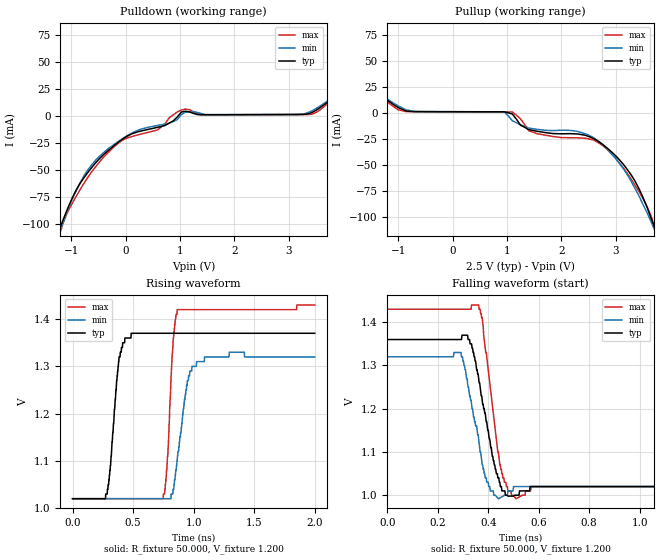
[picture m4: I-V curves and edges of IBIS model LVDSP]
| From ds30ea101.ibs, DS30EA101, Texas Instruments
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|   Model LVDSP
[Model]  LVDSP
Model_type Output
Polarity   Non-Inverting
Vmeas =  1.2V
Rref =   50.0000
Vref =   1.20V
C_comp   417fF   403fF   425fF
[Temperature Range]   25.0000   85.0000   -40.0000
[Voltage Range]   2.5000V   2.3750V   2.6250V
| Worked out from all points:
|   slope of the pulldown table from 0 to 0.375 V, typ, clamps not added: 55.7 ohm
|   slope of the pullup table from 0 to 0.375 V, typ, clamps not added: 8.04 kohm
|   rising waveform, R_fixture 50.000, V_fixture 1.200: 20-80 % time 66ps typ, 94ps min, 47.2ps max; typ from 1.02 V to 1.37 V
|   falling waveform, R_fixture 50.000, V_fixture 1.200: 20-80 % time 64.8ps typ, 56ps min, 51.2ps max; typ from 1.36 V to 1.02 V
[Pulldown]
|Voltage   I(typ)   I(min)   I(max)
-2.5V     -573mA     -566mA     -612mA
-1.225V   -106mA     -109mA     -111mA
-925mV    -69.8mA    -70.7mA    -75.7mA
-700mV    -52.5mA    -50mA      -57mA
-475mV    -39.1mA    -37mA      -42.1mA
-100mV    -22.9mA    -22.3mA    -23.7mA
575mV     -10.5mA    -8.8mA     -13mA
1.025V    3.82mA     1.52mA     5.6mA
3.2V      1.52mA     1.62mA     1.43mA
3.5V      5.37mA     7mA        3.26mA
4.025V    25.9mA     25.5mA     26.5mA
5V        72.8mA     66.5mA     81.9mA
[Pullup]
|Voltage   I(typ)   I(min)   I(max)
-2.5V     72.79mA    66.54mA    81.87mA
-1V       5.372mA    6.997mA    3.261mA
-700mV    1.519mA    1.612mA    1.433mA
950mV     1.29mA     1.332mA    1.182mA
1.1V      -808.5uA   -7.312mA   1.164mA
1.4V      -15.8mA    -14.32mA   -16.88mA
2.45V     -21.31mA   -19.9mA    -24.13mA
2.75V     -29.63mA   -29.55mA   -30.62mA
3.2V      -53.08mA   -57.94mA   -56.71mA
3.5V      -80.59mA   -87.38mA   -81.84mA
3.73V     -111.6mA   -113.6mA   -111.5mA
5V        -569.3mA   -565mA     -608.3mA
[Ramp]
| variable   typ   min   max
dV/dt_r   211.801m/65.502p   201.598m/87.621p   224.397m/48.781p
dV/dt_f   209.399m/58.418p   193.803m/65.933p   224.396m/46.560p
R_load = 50.00
[Rising Waveform]
R_fixture = 50.000
V_fixture = 1.200
V_fixture_min = 1.100
V_fixture_max = 1.300
|  time   V(typ)   V(min)   V(max)
0s        1.02V      1.02V      1.02V
286ps     1.03V      1.02V      1.02V
384ps     1.32V      1.02V      1.02V
484ps     1.37V      1.02V      1.02V
760ps     1.37V      1.02V      1.03V
832ps     1.37V      1.04V      1.36V
864ps     1.37V      1.1V       1.42V
948ps     1.37V      1.27V      1.42V
1.024ns   1.37V      1.31V      1.42V
2ns       1.37V      1.32V      1.43V
[Falling Waveform]
R_fixture = 50.000
V_fixture = 1.200
V_fixture_min = 1.100
V_fixture_max = 1.300
|  time   V(typ)   V(min)   V(max)
0s        1.36V      1.32V      1.43V
292ps     1.36V      1.33V      1.43V
334ps     1.35V      1.21V      1.44V
362ps     1.27V      1.13V      1.44V
376ps     1.22V      1.07V      1.41V
394ps     1.17V      1.03V      1.32V
446ps     1.03V      994mV      1.07V
510ps     1V         1.02V      992mV
570ps     1.02V      1.02V      1.02V
2ns       1.02V      1.02V      1.02V
